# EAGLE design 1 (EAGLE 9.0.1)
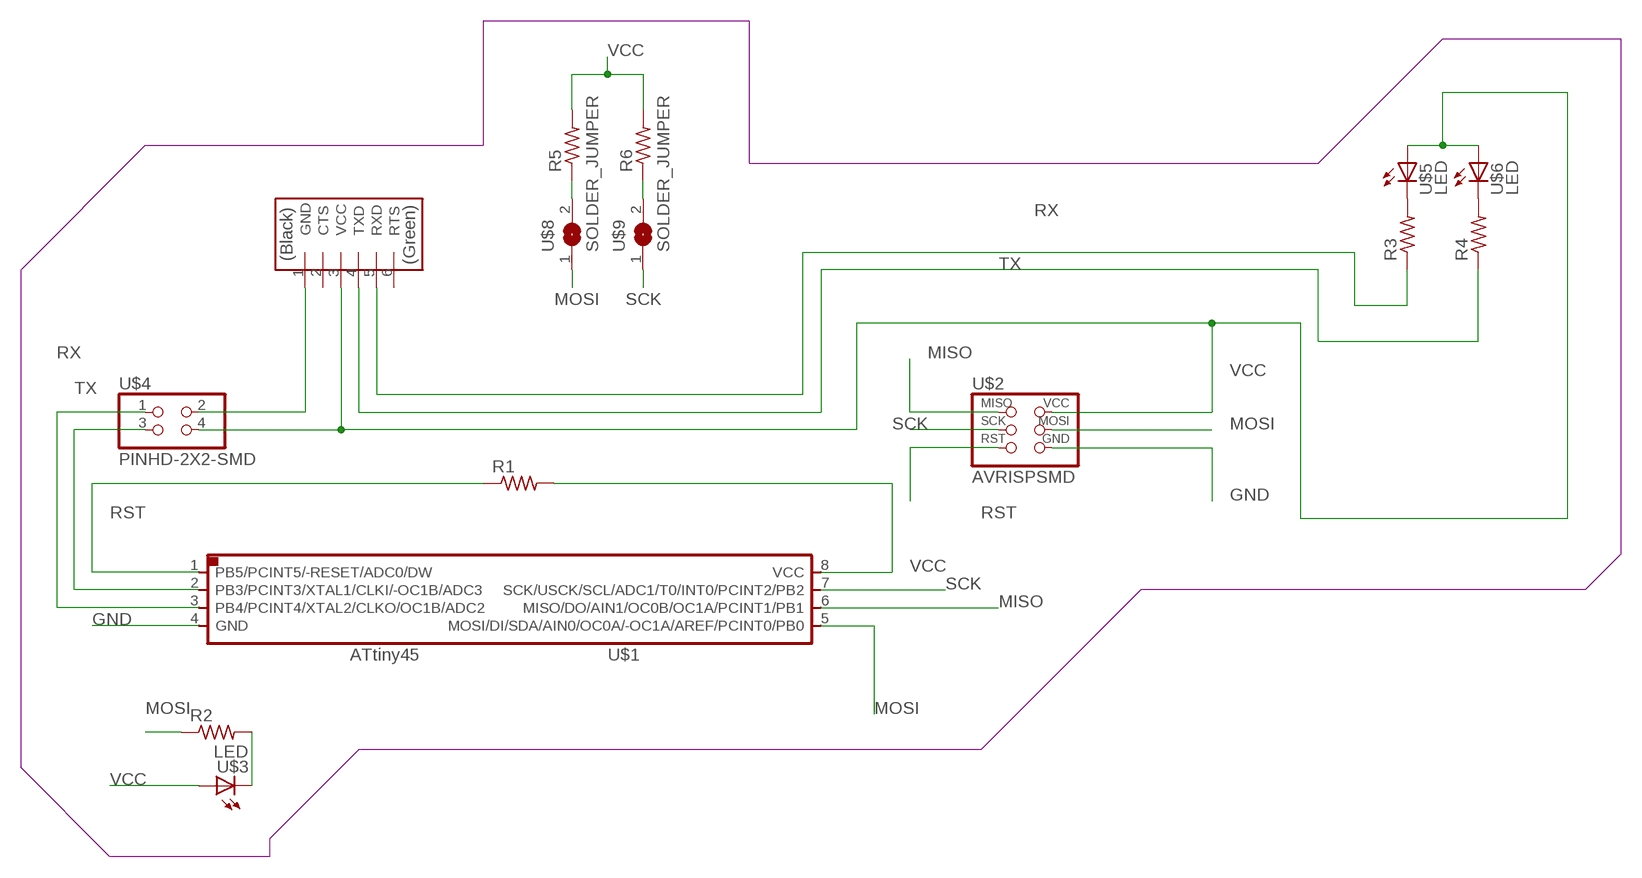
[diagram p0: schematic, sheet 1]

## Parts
R1  RES-US1206  [R1206]
R2  RES-US1206  [R1206]
R3  RES-US1206  [R1206]
R4  RES-US1206  [R1206]
R5  RES-US1206  [R1206]
R6  RES-US1206  [R1206]
U$1  ATTINY45SI  [SOIC8]
U$2  AVRISPSMD  [2X03SMD]
U$3  LED  [LED1206]
U$4  PINHD-2X2-SMD  [2X02SMD]
U$5  LED  [LED1206]
U$6  LED  [LED1206]
U$8  SOLDER_JUMPER  [SJFAB]
U$9  SOLDER_JUMPER  [SJFAB]
U$10  FTDI-SMD-HEADER  [1X06SMD]

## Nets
GND: U$1.4(GND) U$2.6(GND) U$4.2 U$10.1(GND)
MISO: U$1.6(MISO/DO/AIN1/OC0B/OC1A/PCINT1/PB1) U$2.1(MISO)
MOSI: R2.1 U$1.5(MOSI/DI/SDA/AIN0/OC0A/-OC1A/AREF/PCINT0/PB0) U$2.4(MOSI) U$8.1
N$1: R3.2 U$5.2(C)
N$2: R4.2 U$6.2(C)
N$3: R2.2 U$3.2(C)
N$4: R5.1 U$8.2
N$5: R6.1 U$9.2
RST: R1.1 U$1.1(PB5/PCINT5/-RESET/ADC0/DW) U$2.5(RST)
RX: R3.1 U$1.3(PB4/PCINT4/XTAL2/CLKO/OC1B/ADC2) U$4.1 U$10.5(RXD)
SCK: U$1.7(SCK/USCK/SCL/ADC1/T0/INT0/PCINT2/PB2) U$2.3(SCK) U$9.1
TX: R4.1 U$1.2(PB3/PCINT3/XTAL1/CLKI/-OC1B/ADC3) U$4.3 U$10.4(TXD)
VCC: R1.2 R5.2 R6.2 U$1.8(VCC) U$2.2(VCC) U$3.1(A) U$4.4 U$5.1(A) U$6.1(A) U$10.3(VCC)
Unconnected: U$10.2(CTS) U$10.6(RTS)

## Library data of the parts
R1-R6 = fab:RES-US: Resistor (US Symbol)
U$1 = fab:ATTINY45
U$2 = fab:AVRISP
U$3 U$5 U$6 = fab:LED: LED
U$4 = fab:PINHD-2X2-SMD
U$8 U$9 = fab:SOLDER_JUMPER
U$10 = fab:FTDI-SMD-HEADER

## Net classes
0 default: width 0.508 mm, clearance 0.254 mm

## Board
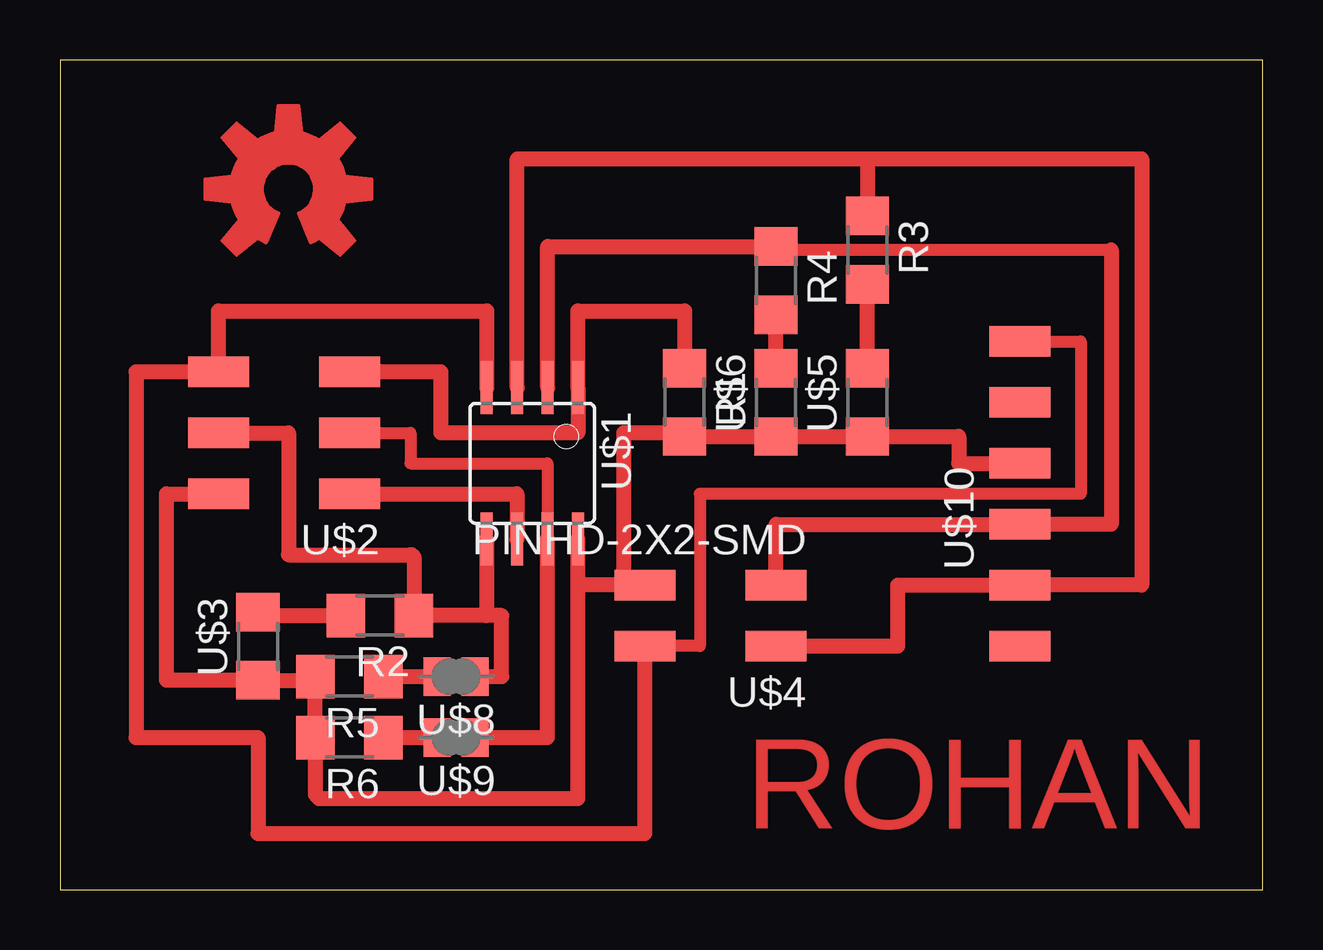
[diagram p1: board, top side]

Size 50.14 x 34.59 mm. Coordinates in mm from the lower left corner, seen from the top.
Outline: 0,0 50.14,0 50.14,34.59 0,34.59 0,0
Copper layers (1*16): Top 0.035mm / dielectric 1.5mm / Bottom 0.035mm
Design rules "default *": minimum track width 6mil, minimum drill 0.35mm, track to track 6mil, track to pad 6mil, pad to pad 6mil, via to via 6mil, smd to smd 6mil, copper to edge 80mil, drill to drill 6mil, minimum pad ring 10mil, minimum via ring 8mil, stop-mask expansion 4mil, vias tented up to drill 0mil, thermal gap 10mil

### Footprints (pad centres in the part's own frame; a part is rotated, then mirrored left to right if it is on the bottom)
R1206 = smd 1.6 x 1.803: 1 -1.422,0; 2 1.422,0
SOIC8 = smd 0.5 x 2.2: 1 -1.905,-3.154; 2 -0.645,-3.154; 3 0.625,-3.154; 4 1.895,-3.154; 5 1.905,3.154; 6 0.635,3.154; 7 -0.635,3.154; 8 -1.905,3.154
2X03SMD = smd 2.54 x 1.27: 1 -2.54,2.54; 2 2.92,2.54; 3 -2.54,0; 4 2.92,0; 5 -2.54,-2.54; 6 2.92,-2.54
LED1206 = smd 1.6 x 1.803: 1 -1.422,0; 2 1.422,0
2X02SMD = smd 2.54 x 1.27: 1 -2.54,1.27; 2 2.92,1.27; 3 -2.54,-1.27; 4 2.92,-1.27
SJFAB = smd 1.118 x 1.6: 1 -0.787,0; 2 0.787,0
1X06SMD = smd 2.54 x 1.27: 1 0,6.35; 2 0,3.81; 3 0,1.27; 4 0,-1.27; 5 0,-3.81; 6 0,-6.35

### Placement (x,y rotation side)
R1  26.04,20.32 270 top
R2  13.34,11.43 180 top
R3  33.66,26.67 270 top
R4  29.84,25.4 270 top
R5  12.07,8.89 180 top
R6  12.07,6.35 180 top
U$1  19.68,17.78 180 top
U$2  9.53,19.05 180 top
U$3  8.26,10.16 90 top
U$4  27.3,11.43 180 top
U$5  33.66,20.32 90 top
U$6  29.84,20.32 90 top
U$7  [OSHW-LOGO-L_COPPER]  9.53,29.21 0 top
U$8  16.51,8.89 180 top
U$9  16.51,6.35 180 top
U$10  40,16.51 0 top

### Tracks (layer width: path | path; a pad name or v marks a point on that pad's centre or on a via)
GND
  Top 0.508: 24.77,10.16 U$4.2 26.67,10.16 26.67,16.51 42.55,16.51 42.55,22.86 U$10.1
  Top 0.635: 6.35,21.59 U$2.6 | U$2.6 3.17,21.59 3.17,6.35 8.26,6.35 8.26,2.35 24.38,2.35 U$4.2 | U$2.6 6.6,24.13 17.79,24.13 U$1.4
MISO
  Top 0.635: U$2.1 19.05,16.51 U$1.6
MOSI
  Top 0.635: U$1.5 17.78,11.43 | 17.78,11.43 R2.1 14.76,13.82 arc90 14.61,13.97 9.53,13.97 9.53,19.05 U$2.4 | U$8.1 18.41,8.89 18.41,11.43 17.78,11.43
N$1
  Top 0.635: U$5.2 R3.2
N$2
  Top 0.635: U$6.2 R4.2
N$3
  Top 0.635: U$3.2 8.26,11.43 R2.2
N$4
  Top 0.635: R5.1 U$8.2
N$5
  Top 0.635: R6.1 U$9.2
RST
  Top 0.635: R1.1 26.04,24.13 21.59,24.13 U$1.1 21.59,19.05 15.88,19.05 15.88,21.59 U$2.5
RX
  Top 0.635: U$1.3 19.06,30.48 33.66,30.48 | U$4.1 34.92,10.16 34.92,12.7 U$10.5 45.09,12.7 45.09,30.48 33.66,30.48 | 33.66,30.48 R3.1
SCK
  Top 0.508: U$1.7 20.32,17.78 14.61,17.78 14.61,19.05 U$2.3
  Top 0.635: U$9.1 20.32,6.35 U$1.7
TX
  Top 0.508: 43.81,26.67 29.84,26.67 R4.1
  Top 0.635: U$1.2 20.33,26.82 R4.1 | U$4.3 29.84,15.24 U$10.4 43.81,15.24 43.81,26.67
VCC
  Top 0.635: U$3.1 4.44,8.74 4.44,16.51 U$2.2 | U$3.1 arc-90 8.41,8.89 | U$4.4 23.49,12.7 23.49,19.05 26.04,19.05 R1.2 U$6.1 U$5.1 37.46,18.9 37.46,17.78 U$10.3 40,17.63 | 24.77,12.7 U$4.4 | U$3.1 10.49,8.74 | 10.49,8.74 R5.2 | 10.49,8.74 10.64,8.59 R6.2 10.64,3.96 10.79,3.81 21.59,3.81 21.59,12.7 | 21.59,12.7 U$1.8 | U$4.4 21.59,12.7

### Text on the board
Top: ROHAN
